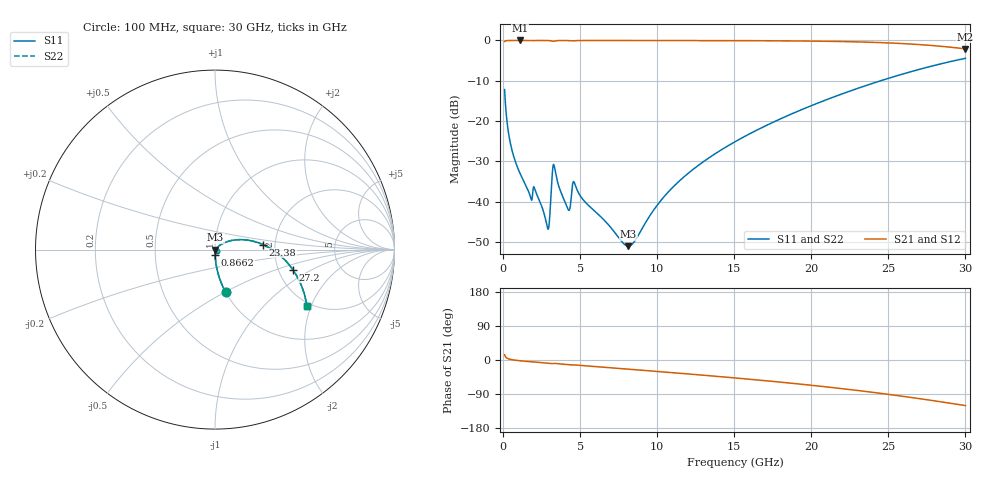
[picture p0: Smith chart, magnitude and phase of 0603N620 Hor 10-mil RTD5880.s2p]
# GHz S MA R 50
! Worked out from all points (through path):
!   3201 points, 100 MHz to 30 GHz, reference 50 ohm
!   highest |S21| = -0.01 dB at 1.09 GHz (marker M1); lowest = -2.1 dB at 30 GHz (marker M2)
!   group delay of S21, straight-line fit = 10.8 ps
!   lowest |S11| = -51.0 dB at 8.126 GHz (marker M3), VSWR 1.01, Z = 50.3 - j0.128 ohm
!   |S11| at or under -10 dB: start of sweep to 24.5 GHz
!   |S22| runs from -51.0 to -4.4 dB; largest |S21 - S12| = 0
!   S11 on the Smith chart (normalised r, x): 100 MHz: 1.00, -0.51; 866.2 MHz: 1.00, -0.06; 23.38 GHz: 1.73, +0.10; 27.2 GHz: 2.40, -0.67; 30 GHz: 1.90, -1.86
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0.1  0.2457 -76.0  0.969 13.9  0.969 13.9  0.2457 -76.0
0.4270312  0.05914 -87.3  0.9977 2.1  0.9977 2.1  0.05914 -87.3
0.8661875  0.02892 -89.3  0.9987 -0.9  0.9987 -0.9  0.02892 -89.3
1.090437  0.02272 -89.6  0.9988 -2.0  0.9988 -2.0  0.02272 -89.6
1.753844  0.01182 -85.0  0.9979 -4.6  0.9979 -4.6  0.01182 -85.0
2.108906  0.0135 -83.6  0.9971 -5.6  0.9971 -5.6  0.0135 -83.6
2.86575  0.004857 -55.6  0.9967 -8.4  0.9967 -8.4  0.004857 -55.6
2.987219  0.005233 -14.5  0.9947 -8.9  0.9947 -8.9  0.005233 -14.5
3.202125  0.02335 -8.6  0.9766 -9.6  0.9766 -9.6  0.02335 -8.6
3.31425  0.02807 -51.4  0.9791 -8.9  0.9791 -8.9  0.02807 -51.4
4.192563  0.008261 -72.6  0.9958 -12.2  0.9958 -12.2  0.008261 -72.6
4.613031  0.01748 -69.6  0.9902 -13.0  0.9902 -13.0  0.01748 -69.6
5.089563  0.01124 -88.9  0.9968 -14.6  0.9968 -14.6  0.01124 -88.9
8.126281  0.002817 -26.9  0.9971 -24.2  0.9971 -24.2  0.002817 -26.9
10.06978  0.009439 39.8  0.9966 -30.4  0.9966 -30.4  0.009439 39.8
12.12541  0.02347 43.8  0.9959 -37.2  0.9959 -37.2  0.02347 43.8
15.05  0.05544 38.1  0.9938 -47.3  0.9938 -47.3  0.05544 38.1
20.03956  0.1564 20.8  0.981 -66.8  0.981 -66.8  0.1564 20.8
23.37528  0.2688 6.0  0.9546 -82.3  0.9546 -82.3  0.2688 6.0
25.01978  0.3396 -2.3  0.9309 -90.8  0.9309 -90.8  0.3396 -2.3
27.19687  0.4476 -14.4  0.8829 -103.0  0.8829 -103.0  0.4476 -14.4
30  0.6002 -31.5  0.7861 -120.2  0.7861 -120.2  0.6002 -31.5
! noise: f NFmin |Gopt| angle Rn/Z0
0.1  0.0002899  0.9178  0.3542  0.0007791
3.417  0.00873  0.9075  10.26  0.02055
6.743  0.00619  0.7634  20.17  0.005152
10.06  0.008355  0.744  29.87  0.006127
13.39  0.01072  0.7388  39.35  0.007307
16.7  0.01336  0.742  48.54  0.008669
20.03  0.01645  0.7518  57.44  0.01034
23.35  0.02022  0.767  66.02  0.0125
26.67  0.02505  0.787  74.33  0.01549
30  0.03155  0.8112  82.39  0.0199
